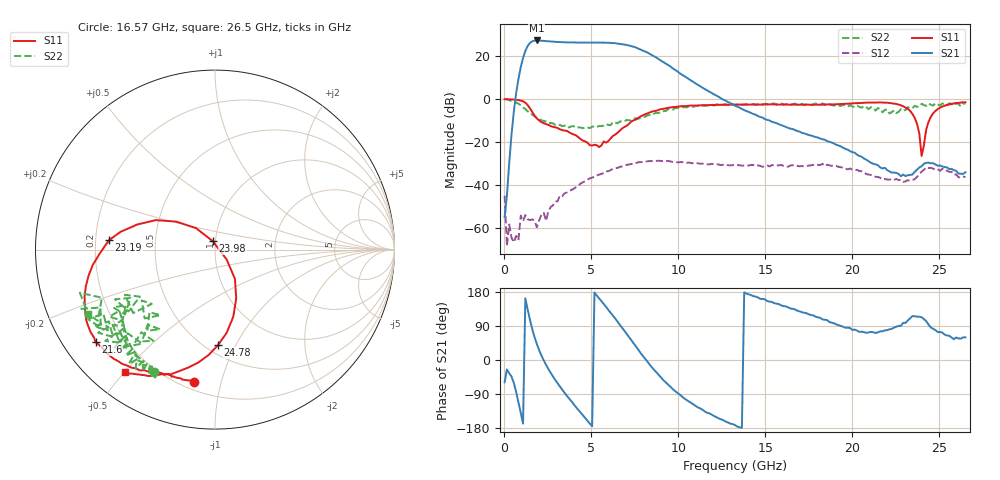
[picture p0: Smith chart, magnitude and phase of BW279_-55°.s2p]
!Agilent Technologies,N5242A,MY52422126,A.09.90.01
!Agilent N5242A: A.09.90.01
!Date: Thursday, January 16, 2014 00:26:51
!Correction: S11(Full 2 Port with power(1,2))
!S21(Full 2 Port with power(1,2))
!S12(Full 2 Port with power(1,2))
!S22(Full 2 Port with power(1,2))
!S2P File: Measurements: S11, S21, S12, S22:
# Hz S  dB  R 50
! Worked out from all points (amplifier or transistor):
!   201 points, 10 MHz to 26.5 GHz, reference 50 ohm
!   highest |S21| = 27.3 dB at 1.864 GHz (marker M1)
!   |S21| within 3 dB of that: 1.31 GHz to 7.455 GHz (6.144 GHz wide, 140 % of centre)
!   unconditionally stable (mu >= 1): 71.46 MHz to end of sweep
!   at 4.381 GHz: K = 2.19, MAG = 26.6 dB, |S12| = -39.2 dB
!   at 13.26 GHz: K = 5.34, MAG = 3.5 dB, |S12| = -30.5 dB
!   at 26.5 GHz: K = 172.65, MAG = -24.2 dB, |S12| = -36.3 dB
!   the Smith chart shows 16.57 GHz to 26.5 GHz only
!   S11 on the Smith chart (normalised r, x): 16.57 GHz: 0.25, -0.83; 21.6 GHz: 0.10, -0.34; 23.19 GHz: 0.26, +0.04; 23.98 GHz: 0.97, +0.09; 24.78 GHz: 0.57, -0.85; 26.5 GHz: 0.11, -0.50
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1e7  -0.04 -1.2  -54.87 -58.9  -44.83 68.7  0.00 -1.4
9.3715e8  -0.63 -146.1  14.81 -139.1  -54.15 166.0  -2.85 -106.4
1.3345e9  -2.73 126.0  24.71 133.5  -55.81 130.1  -5.63 -139.6
1.5994e9  -5.95 61.5  26.89 81.7  -55.88 97.2  -7.14 -157.1
1.8643e9  -8.94 2.6  27.29 42.0  -59.53 97.1  -8.75 -171.7
2.26165e9  -11.20 -63.6  27.08 -1.2  -52.80 106.0  -10.15 169.5
3.05635e9  -13.44 -141.7  26.57 -61.5  -47.47 136.2  -11.91 134.3
3.7186e9  -15.41 174.6  26.37 -101.6  -42.70 117.4  -13.18 110.5
4.5133e9  -19.30 115.1  26.32 -146.0  -38.64 95.2  -13.53 80.2
5.44045e9  -22.26 17.9  26.30 162.6  -35.06 73.6  -12.46 54.7
6.50005e9  -15.65 -101.3  25.85 101.2  -31.92 42.2  -11.23 29.0
7.55965e9  -9.43 167.2  24.00 35.9  -29.71 10.2  -8.93 10.0
8.88415e9  -4.91 74.3  18.49 -40.1  -28.62 -28.7  -6.40 -13.1
1.3255e10  -2.55 -58.0  -3.03 -171.8  -30.52 -110.2  -2.72 -83.6
1.656625e10  -2.52 -98.9  -13.88 135.1  -30.69 -158.1  -2.33 -116.6
1.77583e10  -2.55 -107.2  -17.28 117.7  -30.57 -175.0  -2.44 -125.3
2.159935e10  -1.50 -142.3  -31.73 75.7  -36.52 121.6  -4.55 -144.4
2.212915e10  -1.75 -151.2  -33.58 80.9  -37.45 128.2  -6.66 -139.4
2.318875e10  -4.54 174.9  -35.39 104.3  -37.64 134.5  -3.70 -128.5
2.398345e10  -26.42 104.3  -31.20 112.8  -33.61 142.6  -2.14 -135.8
2.477815e10  -5.49 -88.1  -30.35 78.8  -32.75 98.8  -1.95 -144.6
2.65e10  -1.46 -126.3  -33.96 59.9  -36.29 73.3  -2.02 -153.0
